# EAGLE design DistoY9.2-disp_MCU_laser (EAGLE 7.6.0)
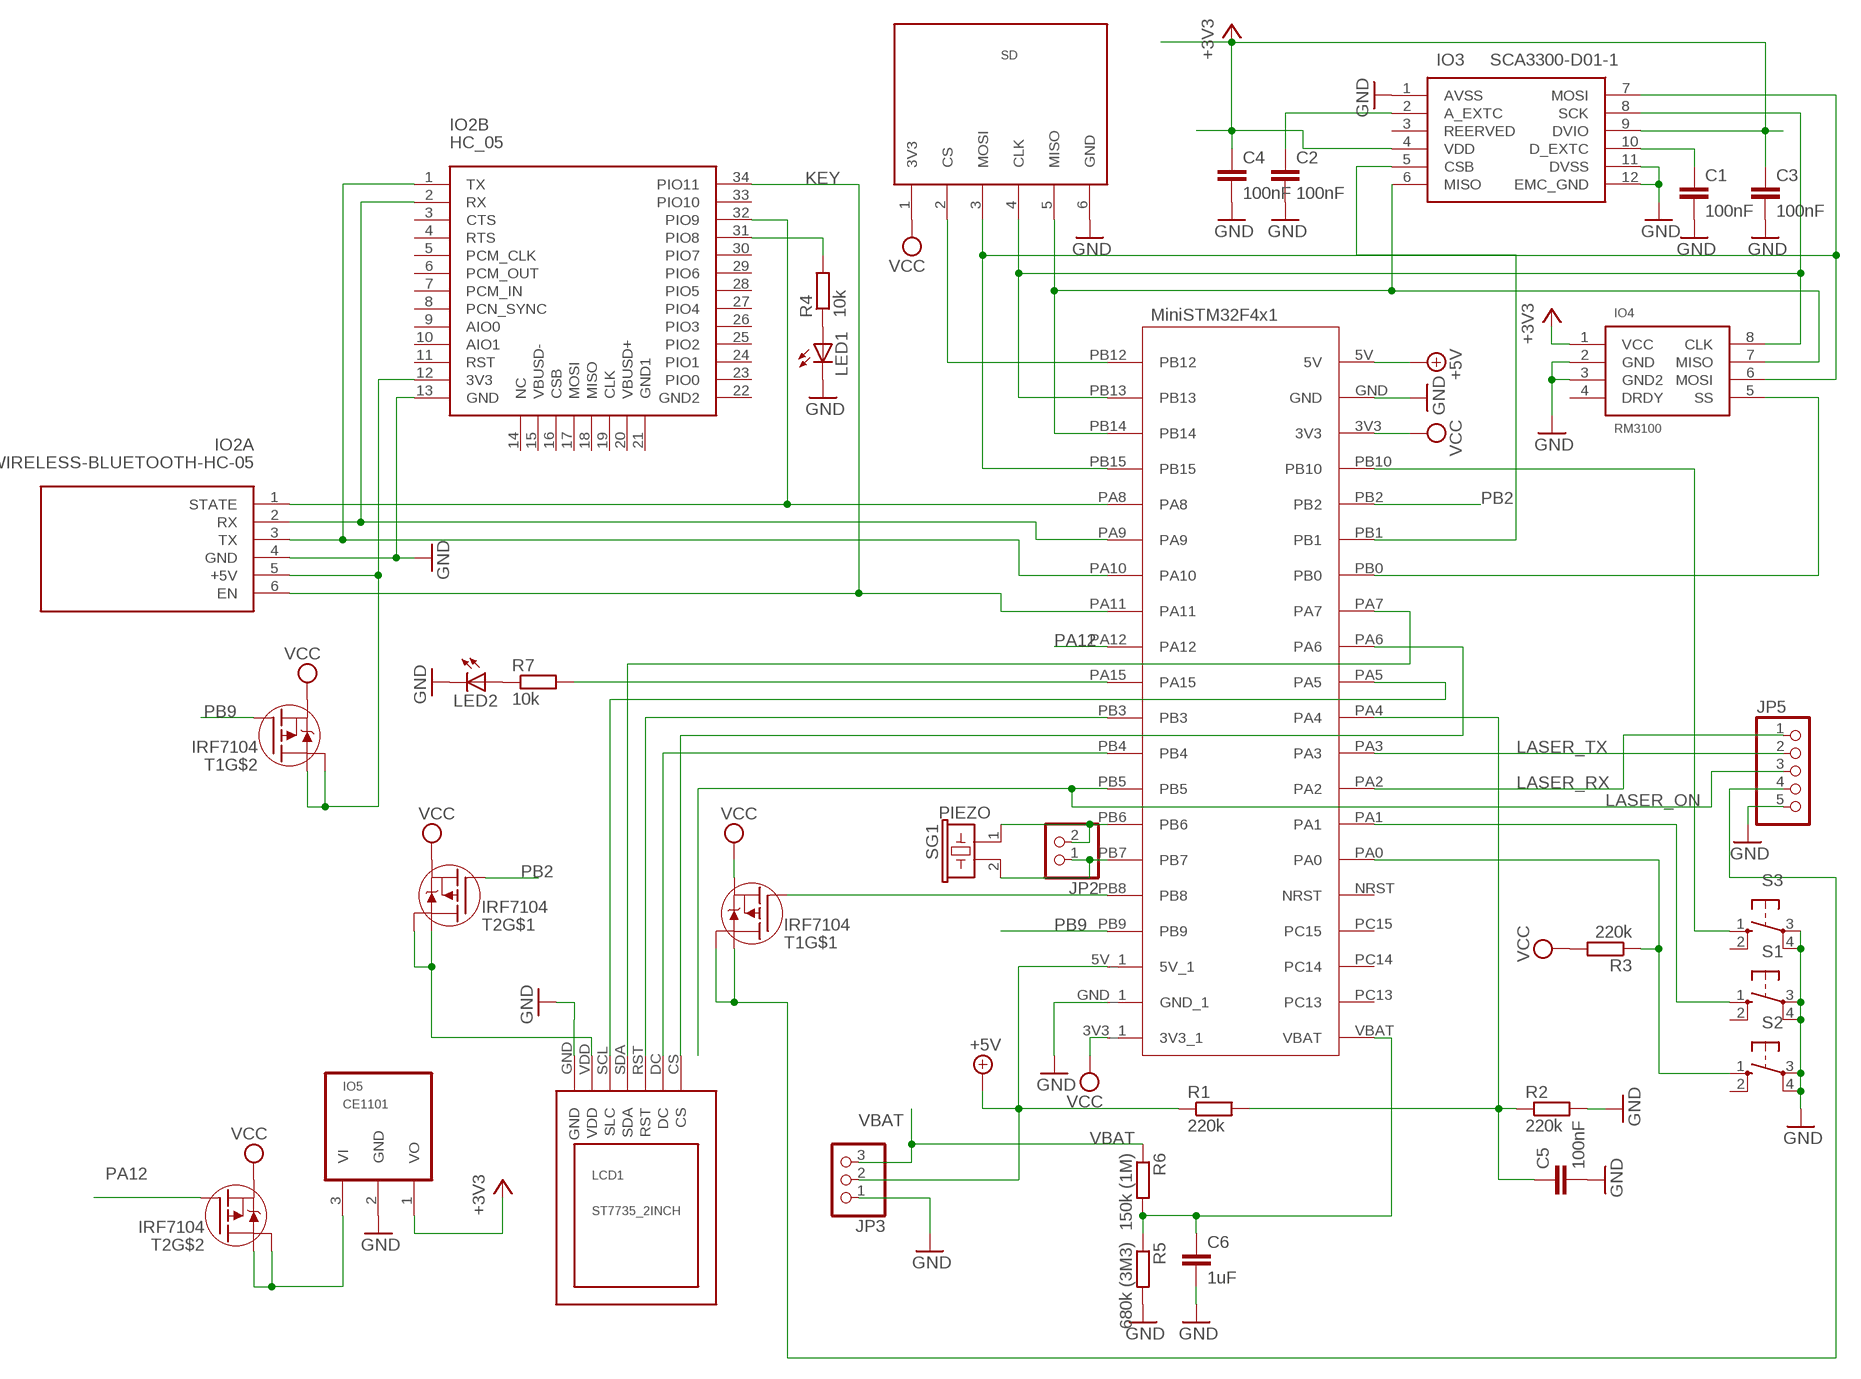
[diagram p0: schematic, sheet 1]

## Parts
C1  100nF  C-EUC0805K  [C0805K]
C2  100nF  C-EUC0805K  [C0805K]
C3  100nF  C-EUC0805K  [C0805K]
C4  100nF  C-EUC0805K  [C0805K]
C5  100nF  C-EUC0805K  [C0805K]
C6  1uF  C-EUC0805K  [C0805K]
IO2A  WIRELESS-BLUETOOTH-HC-05  [WIRELESS-BLUETOOTH-HC-05]
IO2B  HC_05  [BLUETOOTH_SMD]
IO3  SCA3300-D01-1  [SCA3300]
IO4  RM3100  [RM3100]
IO5  CE1101  [CE1101]
JP2  PINHD-1X2/90  [1X02/90]
JP3  PINHD-1X3/90  [1X03/90]
JP5  PINHD-1X5/90  [1X05/90]
LCD1  ST7735_2INCH  [7735_2INCH]
LED1  LEDCHIPLED_0805  [CHIPLED_0805]
LED2  LEDCHIPLED_0805  [CHIPLED_0805]
R1  220k  R-EU_M0805  [M0805]
R2  220k  R-EU_M0805  [M0805]
R3  220k  R-EU_M0805  [M0805]
R4  10k  R-EU_R0805  [R0805]
R5  680k (3M3)  R-EU_M0805  [M0805]
R6  150k (1M)  R-EU_M0805  [M0805]
R7  10k  R-EU_R0805  [R0805]
S1  10-XX  [B3F-10XX]
S2  10-XX  [B3F-10XX]
S3  10-XX  [B3F-10XX]
SD  SD  [SD]
SG1  PIEZO  B/C11L  [B/C11L]
T1  IRF7104  [SO8-2]
T2  IRF7104  [SO8-2]
U$1  STM32F401  [STM32F401]

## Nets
+3V3: C3.1 C4.1 IO3.4(VDD) IO3.9(DVIO) IO4.1(VCC) IO5.1(VO)
+5V: JP3.2 R1.1 U$1.5V U$1.5V_1
GND: C1.2 C2.2 C3.2 C4.2 C5.2 C6.2 IO2A.4(GND) IO2B.13(GND) IO3.1(AVSS) IO3.11(DVSS) IO3.12(EMC_GND) IO4.2(GND) IO4.3(GND2) IO5.2(GND) JP3.1 JP5.5 LCD1.GND LED1.C LED2.C R2.2 R5.2 S1.3(P) S1.4(P1) S2.3(P) S2.4(P1) S3.3(P) S3.4(P1) SD.6(GND) U$1.GND U$1.GND_1
KEY: IO2A.6(EN) IO2B.34(PIO11) U$1.PA11
LASER_ON: JP5.3 U$1.PB5
LASER_RX: JP5.1 U$1.PA2
LASER_TX: JP5.2 U$1.PA3
N$1: IO2A.2(RX) IO2B.2(RX) U$1.PA9
N$2: IO2A.3(TX) IO2B.1(TX) U$1.PA10
N$3: S3.1(S) U$1.PB10
N$4: IO2A.5(+5V) IO2B.12(3V3) T1.5(D) T1.6(D)
N$5: LCD1.SDA U$1.PA7
N$6: LCD1.SCL(SLC) U$1.PA5
N$7: IO2A.1(STATE) IO2B.32(PIO9) U$1.PA8
N$9: C6.1 R5.1 R6.2 U$1.VBAT
N$10: S1.1(S) U$1.PA1
N$11: R3.1 S2.1(S) U$1.PA0
N$12: LCD1.DC U$1.PB4
N$13: LCD1.RST U$1.PB3
N$14: LED2.A R7.1
N$15: T1.2(G) U$1.PB8
N$16: JP5.4 T1.7(D) T1.8(D)
N$17: IO3.6(MISO) IO4.7(MISO) SD.5(MISO) U$1.PB14
N$19: LED1.A R4.1
N$20: IO3.7(MOSI) IO4.6(MOSI) SD.3(MOSI) U$1.PB15
N$21: IO2B.31(PIO8) R4.2
N$22: IO3.8(SCK) IO4.8(CLK) SD.4(CLK) U$1.PB13
N$23: SD.2(CS) U$1.PB12
N$24: C2.1 IO3.2(A_EXTC)
N$25: C1.1 IO3.10(D_EXTC)
N$26: IO4.5(SS) U$1.PB0
N$27: LCD1.VDD T2.7(D) T2.8(D)
N$28: LCD1.CS U$1.PA6
N$29: IO3.5(CSB) U$1.PB1
N$31: JP2.2 SG1.1 U$1.PB6
N$32: JP2.1 SG1.2 U$1.PB7
N$33: C5.1 R1.2 R2.1 U$1.PA4
N$34: R7.2 U$1.PA15
N$35: IO5.3(VI) T2.5(D) T2.6(D)
PA12: T2.4(G) U$1.PA12
PB2: T2.2(G) U$1.PB2
PB9: T1.4(G) U$1.PB9
VBAT: JP3.3 R6.1
VCC: R3.2 SD.1(3V3) T1.1(S) T1.3(S) T2.1(S) T2.3(S) U$1.3V3 U$1.3V3_1
Unconnected: IO2B.3(CTS) IO2B.4(RTS) IO2B.5(PCM_CLK) IO2B.6(PCM_OUT) IO2B.7(PCM_IN) IO2B.8(PCN_SYNC) IO2B.9(AIO0) IO2B.10(AIO1) IO2B.11(RST) IO2B.14(NC) IO2B.15(VBUSD-) IO2B.16(CSB) IO2B.17(MOSI) IO2B.18(MISO) IO2B.19(CLK) IO2B.20(VBUSD+) IO2B.21(GND1) IO2B.22(GND2) IO2B.23(PIO0) IO2B.24(PIO1) IO2B.25(PIO2) IO2B.26(PIO3) IO2B.27(PIO4) IO2B.28(PIO5) IO2B.29(PIO6) IO2B.30(PIO7) IO2B.33(PIO10) IO3.3(REERVED) IO4.4(DRDY) S1.2(S1) S2.2(S1) S3.2(S1) U$1.NRST U$1.PC13 U$1.PC14 U$1.PC15

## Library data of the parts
C1-C6 = rcl:C-EU: CAPACITOR, European symbol
IO2A = diy-modules:WIRELESS-BLUETOOTH-HC-05: Bluetooth Transceiver Module based on HC-05 board Tutorial is available here: https://arduino-info.wikispaces.com/BlueTooth-HC05-HC06-Modules-How-To Click here to find device on ebay.com
IO2B = SerialPortBluetooth:HC_05
IO3 = SCA3300-D01-1:SCA3300-D01-1: Murata SCA3300-D01-1, 3-Axis Accelerometer, +/-1.5 +/-6g, 3 3.6 V, SPI, DFL/SMD 12-Pin Source: Datasheet Check availability; AVAILABILITY: In Stock; DESCRIPTION: Accelerometer X, Y, Z Axis ±1.5g, 3g, 6g - -; MF: Murata Electronics; MP: SCA3300-D01-1; PACKAGE: Nonstandard Murata; PRICE: None; PURCHASE-URL: https://pricing.snapeda.com/search/part/SCA3300-D01-1/?ref=eda
IO4 = SCA3300-D01-1:RM3100
IO5 = SCA3300-D01-1:CE1101
JP2 = pinhead:PINHD-1X2: PIN HEADER
JP3 = pinhead:PINHD-1X3: PIN HEADER
JP5 = pinhead:PINHD-1X5: PIN HEADER
LCD1 = st7735:ST7735_2INCH
LED1 LED2 = led:LED: LED
R1-R7 = rcl:R-EU_: RESISTOR, European symbol
S1-S3 = switch-omron:10-XX: OMRON SWITCH; MPN: B3F-1000; OC_FARNELL: 176432; OC_NEWARK: 36M3542
SD = memory:SD
SG1 = buzzer:B/C11L: BUZZER; OC_FARNELL: unknown; OC_NEWARK: unknown
T1 T2 = irf-2:IRF7104: HEXFET® Power MOSFET Adavanced Process Technology Ultra Low On-Resistance Dual P-Channel MOSFET Surface Mount Available in Tape & Reel Dynamic dv/dt Rating Fast Switching Please connect both Drain-Pins of each FET for thermal Reasons! (Pin 5 with Pin 6, 7 with 8)
U$1 = MiniSTM32F4x1_EAGLE:STM32F401

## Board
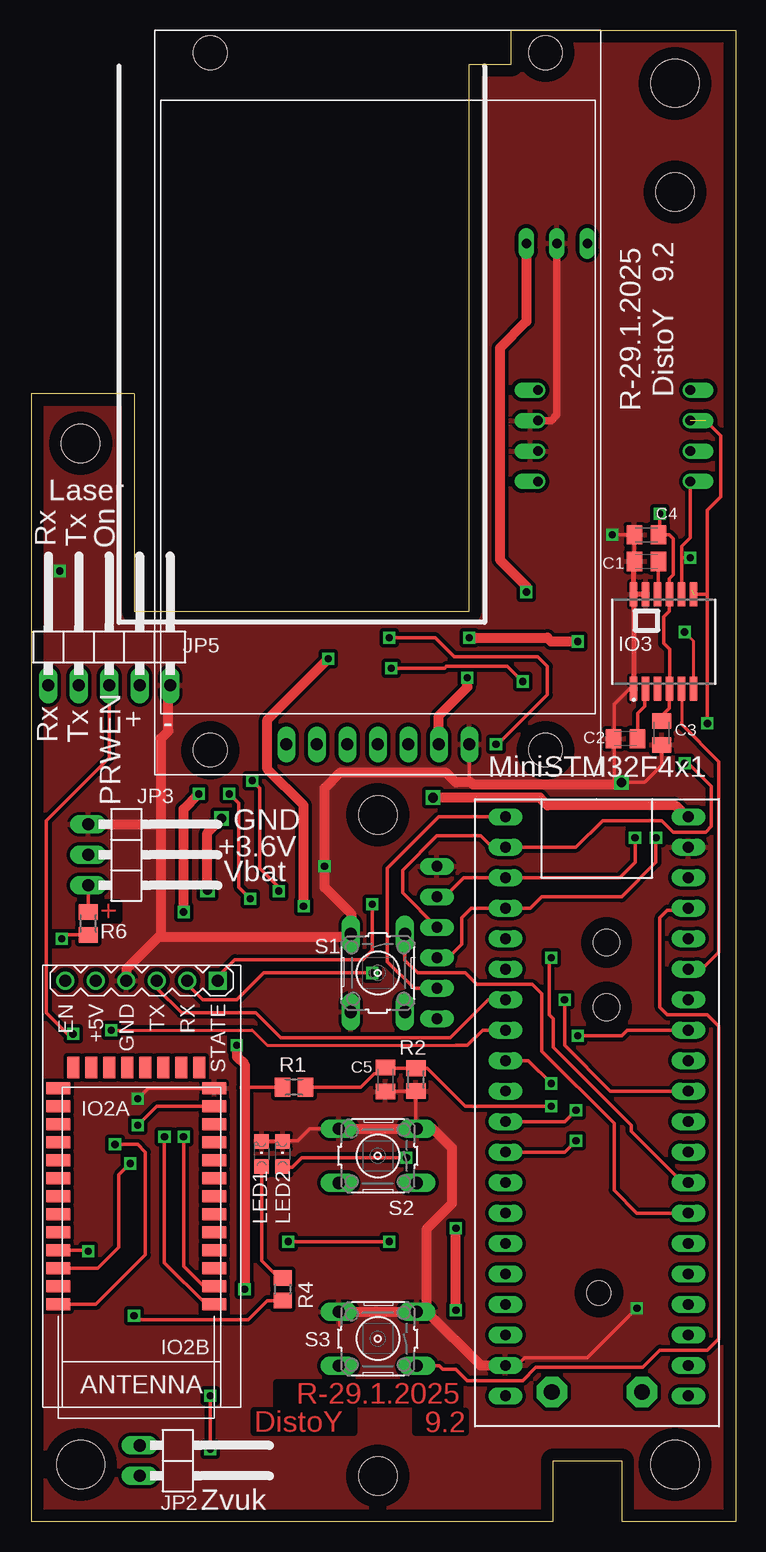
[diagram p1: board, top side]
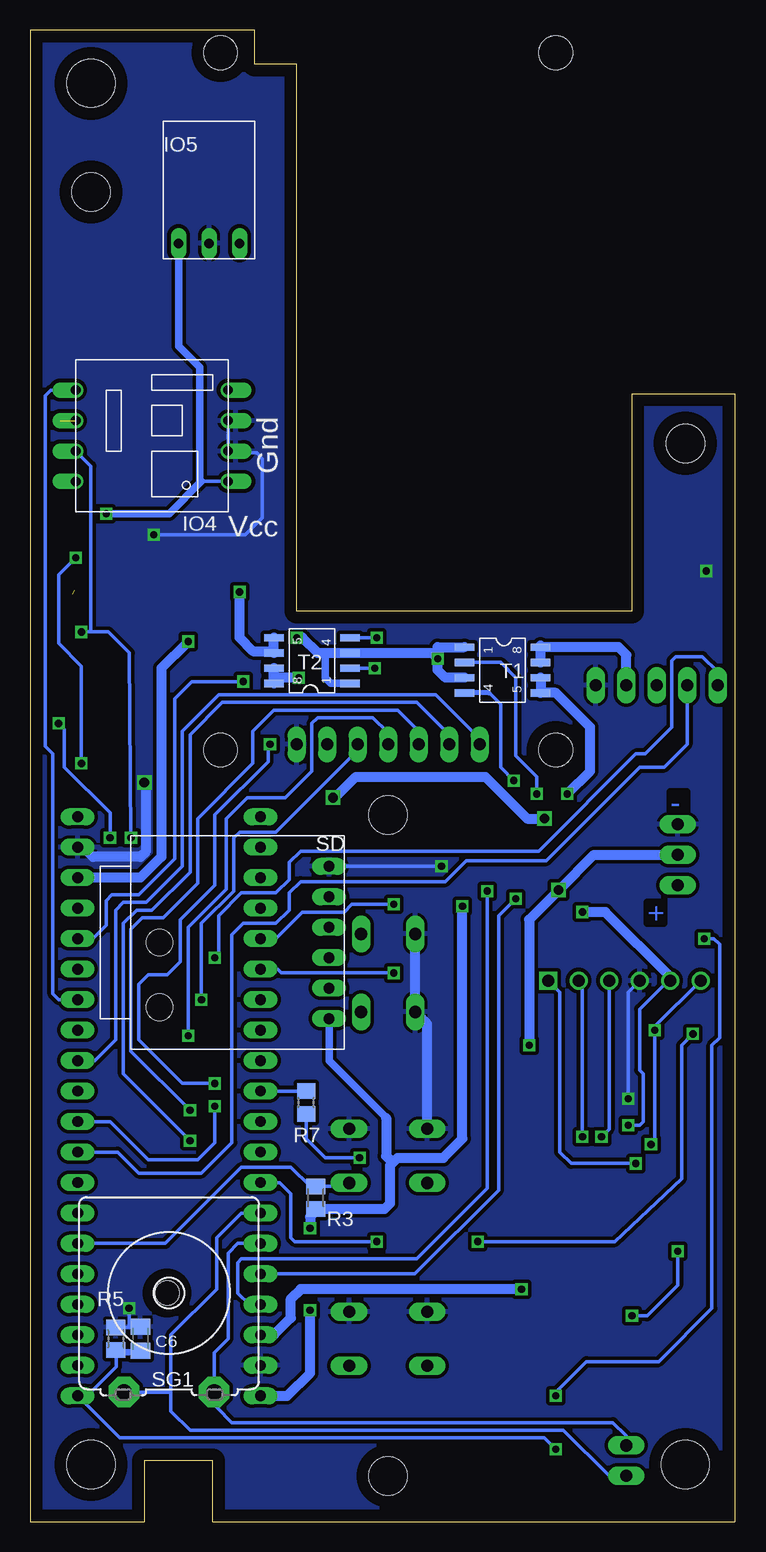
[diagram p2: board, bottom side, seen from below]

Size 58.74 x 124.3 mm. Coordinates in mm from the lower left corner, seen from the top.
Outline: 0,93.98 0,0 43.5,0 43.5,5.08 49.21,5.08 49.21,0 58.74,0 58.74,124.3 40.01,124.3 40.01,121.44 36.51,121.44 36.51,75.88 8.57,75.88 8.57,93.98 0,93.98
Copper layers (1*16): Top 0.035mm / dielectric 1.5mm / Bottom 0.035mm
Design rules "default": minimum track width 10mil, minimum drill 24mil, track to track 8mil, track to pad 8mil, pad to pad 8mil, via to via 8mil, smd to smd 8mil, copper to edge 40mil, drill to drill 8mil, minimum pad ring 10mil, minimum via ring 8mil, stop-mask expansion 4mil, vias tented up to drill 0mil, thermal gap 10mil
Holes 4 mm at 53.66,4.76 4.13,4.76 53.66,119.86
Holes 2 mm at 47.31,19.05
Holes 3.2 mm at 28.89,58.9 28.89,3.81 53.66,110.81 4.13,89.85
Holes 2.2 mm at 47.94,48.26 47.94,42.86

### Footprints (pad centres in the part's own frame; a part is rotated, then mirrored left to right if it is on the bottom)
C0805K = smd 1.3 x 1.6: 1 -1,0; 2 1,0
WIRELESS-BLUETOOTH-HC-05 = drill 1 square: 1 -6.35,-17.145 | drill 1: 2 -3.81,-17.145; 3 -1.27,-17.145; 4 1.27,-17.145; 5 3.81,-17.145; 6 6.35,-17.145
BLUETOOTH_SMD = smd 2 x 1: 1 0,0; 2 0,-1.5; 3 0,-3; 4 0,-4.5; 5 0,-6; 6 0,-7.5; 7 0,-9; 8 0,-10.5; 9 0,-12; 10 0,-13.5; 11 0,-15; 12 0,-16.5; 13 0,-18; 22 13,-18; 23 13,-16.5; 24 13,-15; 25 13,-13.5; 26 13,-12; 27 13,-10.5; 28 13,-9; 29 13,-7.5; 30 13,-6; 31 13,-4.5; 32 13,-3; 33 13,-1.5; 34 13,0 | smd 1 x 1.8: 14 1.25,-19.75; 15 2.75,-19.75; 16 4.25,-19.75; 17 5.75,-19.75; 18 7.25,-19.75; 19 8.75,-19.75; 20 10.25,-19.75; 21 11.75,-19.75
SCA3300 = smd 0.61 x 2: 1 -2.5,-3.935; 2 -1.5,-3.935; 3 -0.5,-3.935; 4 0.5,-3.935; 5 1.5,-3.935; 6 2.5,-3.935; 7 2.5,3.935; 8 1.5,3.935; 9 0.5,3.935; 10 -0.5,3.935; 11 -1.5,3.935; 12 -2.5,3.935
RM3100 = drill 0.8 offset: 1 -6.35,2.54; 2 -6.35,0; 3 -6.35,-2.54; 4 -6.35,-5.08; 5 6.35,-5.08; 6 6.35,-2.54; 7 6.35,0; 8 6.35,2.54
CE1101 = drill 0.8 long: 1 -2.54,-3.81; 2 0,-3.81; 3 2.54,-3.81
1X02/90 = drill 1.016 long: 1 -1.27,-3.81; 2 1.27,-3.81
1X03/90 = drill 1.016 long: 1 -2.54,-3.81; 2 0,-3.81; 3 2.54,-3.81
1X05/90 = drill 1.016 long: 1 -5.08,-3.81; 2 -2.54,-3.81; 3 0,-3.81; 4 2.54,-3.81; 5 5.08,-3.81
7735_2INCH = drill 1 long: CS 7.62,24.765; DC 5.08,24.765; GND -7.62,24.765; RST 2.54,24.765; SCL -2.54,24.765; SDA 0,24.765; VDD -5.08,24.765 | hole 2.8: 13.97,25.241; -13.97,25.241; 13.97,-32.861; -13.97,-32.861
CHIPLED_0805 = smd 1.2 x 1.2: A 0,-1.05; C 0,1.05
M0805 = smd 1.3 x 1.6: 1 -0.95,0; 2 0.95,0
R0805 = smd 1.3 x 1.5: 1 -0.95,0; 2 0.95,0
B3F-10XX = drill 1.016 long: 1 -3.251,2.261; 2 3.251,2.261; 3 -3.251,-2.261; 4 3.251,-2.261
SD = drill 0.9 long: 1 -6.35,-6.35; 2 -3.81,-6.35; 3 -1.27,-6.35; 4 1.27,-6.35; 5 3.81,-6.35; 6 6.35,-6.35
B/C11L = drill 1.321 pad 2.54 octagon: 1 -3.759,-8.255; 2 3.759,-8.255
SO8-2 = smd 0.61 x 1.626: 1 -2.54,-2.54; 2 -1.27,-2.54; 3 0,-2.54; 4 1.27,-2.54; 5 1.27,3.81; 6 0,3.81; 7 -1.27,3.81; 8 -2.54,3.81
STM32F401 = drill 0.9 long: 3V3 7.62,21.59; 3V3_1 -7.62,-21.59; 5V 7.62,26.67; 5V_1 -7.62,-16.51; GND 7.62,24.13; GND_1 -7.62,-19.05; NRST 7.62,-11.43; PA0 7.62,-8.89; PA1 7.62,-6.35; PA2 7.62,-3.81; PA3 7.62,-1.27; PA4 7.62,1.27; PA5 7.62,3.81; PA6 7.62,6.35; PA7 7.62,8.89; PA8 -7.62,16.51; PA9 -7.62,13.97; PA10 -7.62,11.43; PA11 -7.62,8.89; PA12 -7.62,6.35; PA15 -7.62,3.81; PB0 7.62,11.43; PB1 7.62,13.97; PB2 7.62,16.51; PB3 -7.62,1.27; PB4 -7.62,-1.27; PB5 -7.62,-3.81; PB6 -7.62,-6.35; PB7 -7.62,-8.89; PB8 -7.62,-11.43; PB9 -7.62,-13.97; PB10 7.62,19.05; PB12 -7.62,26.67; PB13 -7.62,24.13; PB14 -7.62,21.59; PB15 -7.62,19.05; PC13 7.62,-19.05; PC14 7.62,-16.51; PC15 7.62,-13.97; VBAT 7.62,-21.59

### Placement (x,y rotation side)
C1  51.28,80.01 180 top
C2  49.53,65.25 180 top
C3  52.55,65.72 270 top
C4  51.28,82.23 180 top
C5  29.53,36.83 270 top
C6  49.53,15.24 90 bottom
IO2A  9.21,27.94 180 top
IO2B  15.24,18.1 180 top
IO3  52.7,73.34 0 top
IO4  48.58,89.22 180 bottom
IO5  43.81,110.33 0 bottom
JP2  12.86,5.08 270 top
JP3  8.57,55.56 270 top
JP5  6.51,73.5 0 top
LCD1  28.89,89.53 180 top
LED1  19.21,30.64 0 top
LED2  20.95,30.64 0 top
R1  21.91,36.2 0 top
R2  32.07,36.83 270 top
R3  34.92,26.99 270 bottom
R4  20.95,19.37 270 top
R5  51.59,15.24 90 bottom
R6  4.76,49.85 270 top
R7  35.72,34.92 90 bottom
S1  28.89,45.72 270 top
S2  28.89,30.48 180 top
S3  28.89,15.24 180 top
SD  40.16,48.26 90 bottom
SG1  47.15,19.05 0 bottom
T1  20,70.33 270 bottom
T2  34.61,72.39 90 bottom
U$1  47.15,32.07 0 top

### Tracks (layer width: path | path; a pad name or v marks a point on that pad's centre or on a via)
+3V3  (via drill 0.6)
  Top 0.305: C3.1 52.55,67.15 53.18,67.79 53.18,69.38 IO3.4 53.2,72.68 52.7,73.18 52.7,75.41 53.18,75.88 53.18,77.25 IO3.9 53.18,77.3 53.18,78.58 53.5,78.9 53.5,81.92 53.18,82.23 52.39,82.23 | C4.1 52.39,82.23 | 52.39,82.23 v52.39,83.98
  Bottom 0.305: 44.61,96.36 44.61,96.2 | IO4.1 44.45,86.68
  Bottom 0.61: IO5.1 46.35,97.95 44.61,96.2 44.61,86.84 44.45,86.68 47.15,83.98 v52.39,83.98
+5V  (via drill 0.6, 0.8)
  Top 0.305: R1.1 17.78,36.2
  Top 0.813: v17.15,39.69 17.15,38.73 17.78,38.1 17.78,36.2 v17.78,19.37 | U$1.5V 54.61,58.74 53.66,59.69 43.02,59.69 42.39,60.33 v33.5,60.33 | v14.68,52.63 14.68,57.39 v15.88,58.58
  Bottom 0.813: v17.15,39.69 17.15,50.16 v14.68,52.63 11.75,55.56 JP3.2 | U$1.5V_1 38.42,15.56 36.99,16.99 36.99,18.57 36.2,19.37 v17.78,19.37 | v33.5,60.33 33.34,60.33 31.59,62.07 20.8,62.07 17.3,58.58 v15.88,58.58
GND  (via drill 0.6, 0.8)
  Top 0.305: C5.2 29.58,35.88 R2.2 32.07,32.82 S2.3 | IO2B.13 9.74,36.1 v8.89,35.24 | 25.72,16.35 25.72,17.42 S3.4 | IO3.1 49.88,69.41 48.58,68.1 48.58,65.29 | 48.58,65.29 C2.2 | 48.58,65.29 48.58,61.59 | C1.2 C4.2 v48.42,82.23 | LCD1.GND 36.51,61.75 36.67,61.59 | v50.48,17.78 46.35,13.65 41.12,13.65 40.48,13.02 U$1.GND_1 | S2.4 23.22,32.74 22.22,31.75 21.02,31.75 LED2.C LED1.C | v24.45,54.61 24.77,54.61 24.45,54.29 | C3.2 52.55,63.02 51.12,61.59 v49.21,61.59
  Top 0.406: IO3.11 IO3.12 | IO3.12 IO3.1 | IO3.12 50.2,79.94 C1.2
  Top 0.61: IO5.2 43.81,92.23 43.34,91.76 IO4.3
  Top 0.813: S3.4 28.73,17.5 | 28.73,17.5 S3.3 32.7,17.5 | 28.89,17.34 28.73,17.5 | 32.7,17.5 32.98,17.5 37.46,13.02 U$1.GND_1 | 32.7,17.5 32.98,17.78 32.98,24.41 35.08,26.51 35.08,31.11 33.46,32.74 S2.3 S2.4 | 10.8,58.1 10.8,65.25 11.43,65.88 11.43,69.53 JP5.5 | 10.8,48.74 10.64,48.74 7.94,46.04 IO2A.4 | JP3.1 10.8,58.1 | 10.8,58.1 10.8,48.74 | 10.8,48.74 26.4,48.74 S1.3 26.67,49.01 26.67,50.64 24.45,52.86 24.45,54.29 24.45,61.12 25.72,62.39 34.61,62.39 35.4,61.59 36.67,61.59 36.83,61.44 49.05,61.44 v49.21,61.59
  Bottom 0.305: v8.89,35.24 8.89,44.13 IO2A.4 | C6.2 50.43,16.24 R5.2 50.48,16.19 | 50.48,16.19 49.53,16.19 | IO4.3 IO4.2 42.07,89.06 39.85,89.06 39.37,88.58 39.37,83.66 40.8,82.23 v48.42,82.23 | v50.48,17.78 50.48,16.19 | SD.6 v24.45,54.61
  Bottom 0.813: S2.4 25.64,41.48 S1.4 | 26.67,42.43 S1.4 | v49.21,61.59 49.05,60.96 49.05,55.88 49.53,55.4 53.5,55.4 54.13,56.04 54.61,56.04 U$1.GND | S1.4 S1.3
  other vias: 2.38,79.22
  pour Bottom (isolate 0.305): -0.79,124.62 59.21,124.62 59.37,-0.95 -0.64,-0.95
  pour Top (isolate 0.305): -0.48,124.62 59.21,124.62 59.05,-0.64 -0.64,-0.64
KEY  (via drill 0.6)
  Top 0.254: 6.99,40.96 18.41,40.96 19.68,39.69 35.4,39.69
  Top 0.305: IO2B.34 5.4,18.1 9.52,22.23 9.52,30.8 8.89,31.43 v6.99,31.43 | 35.4,39.69 36.35,39.69 37.62,40.96 U$1.PA11 | 6.99,40.96 v6.67,40.96
  Bottom 0.305: v6.99,31.43 6.67,31.75 6.67,40.48 v6.67,40.96 6.67,41.27 IO2A.6
LASER_ON  (via drill 0.6)
  Top 0.305: JP5.3 6.51,63.66 1.27,58.42 1.27,42.39 3.02,40.64 v3.49,40.64 | v29.84,23.34 v21.43,23.34
  Bottom 0.305: U$1.PB5 37.94,28.26 36.99,27.3 36.99,23.65 36.67,23.34 v29.84,23.34 | v21.43,23.34 10,23.34 4.44,28.57 4.44,39.69 v3.49,40.64
LASER_RX  (via drill 0.6)
  Top 0.305: U$1.PA2 54.29,28.26 50.01,32.54 50.01,33.02 43.5,39.53 43.5,41.91 43.18,42.23 43.18,46.83 v43.34,46.99
  Bottom 0.305: 43.34,47.15 v43.34,46.99 43.02,47.31 43.02,50.48 41.12,52.39 38.26,52.39 37.15,53.5 37.15,54.93 36.2,55.88 16.35,55.88 8.25,63.98 7.46,63.98 5.24,66.2 5.24,71.75 4.92,72.07 2.7,72.07 1.43,70.8 JP5.1
LASER_TX
  Bottom 0.305: U$1.PA3 51.44,30.8 49.69,29.05 44.45,29.05 41.91,31.59 41.91,48.9 40.96,49.85 38.26,49.85 37.15,50.96 37.15,52.39 36.2,53.34 24.13,53.34 22.38,55.09 15.72,55.09 7.94,62.87 5.87,62.87 3.97,64.77 JP5.2
N$1  (via drill 0.6)
  Top 0.305: IO2A.2 13.02,44.77 14.29,43.5 17.15,43.5 19.37,45.72 v28.42,45.72 | IO2B.2 14.38,19.6 12.7,21.27 v12.7,32.07
  Bottom 0.305: v12.7,32.07 12.7,44.77 IO2A.2 | v28.42,45.72 37.78,45.72 38.1,46.04 U$1.PA9
N$2  (via drill 0.6)
  Top 0.305: IO2A.3 10.48,44.45 12.54,42.39 18.73,42.39 20.8,40.32 34.92,40.32 38.1,43.5 U$1.PA10 | IO2B.1 14.6,18.1 11.11,21.59 v11.11,32.07
  Bottom 0.305: IO2A.3 10.48,32.7 v11.11,32.07
N$3
  Top 0.305: S3.1 34.01,12.98 34.29,12.7 35.4,12.7 36.35,11.75 40.96,11.75 42.07,12.86 50.96,12.86 52.39,14.29 56.36,14.29 57.31,15.24 57.31,41.27 56.36,42.23 53.02,42.23 52.39,42.86 52.39,50.32 53.02,50.96 54.61,50.96 U$1.PB10
N$4  (via drill 0.6)
  Top 0.305: IO2B.12 10.47,34.6 v8.89,33.02
  Top 0.813: v12.7,50.8 12.7,59.37 v13.97,60.64
  Bottom 0.305: v8.89,33.02 7.94,33.02 7.62,33.34 7.62,37.31 7.94,37.62 7.94,42.7 5.56,45.09 IO2A.5
  Bottom 0.813: v12.7,50.8 10.8,50.8 5.4,45.4 IO2A.5 | v13.97,60.64 12.07,62.55 12.07,66.2 14.92,69.06 T1.5 T1.6
N$5  (via drill 0.6)
  Top 0.305: U$1.PA7 49.69,40.96 49.21,40.48 v45.56,40.48
  Bottom 0.305: v45.56,40.48 45.56,49.53 42.39,52.7 42.39,58.58 40.64,60.33 37.46,60.33 35.24,62.55 35.24,66.52 34.77,66.99 30.16,66.99 28.89,65.72 LCD1.SDA
N$6  (via drill 0.6)
  Top 0.305: v44.45,43.5 44.45,39.69 48.26,35.88 U$1.PA5
  Bottom 0.305: v44.45,43.5 44.45,49.85 41.75,52.55 41.75,56.99 41.27,57.47 38.26,57.47 31.43,64.29 LCD1.SCL
N$7  (via drill 0.6)
  Top 0.305: IO2B.32 5.54,21.1 7.3,22.86 7.3,28.89 v8.25,29.84 | IO2A.1 15.56,45.4 16.99,46.83 27.62,46.83 28.42,47.62 v28.42,51.44
  Bottom 0.305: v8.25,29.84 13.65,29.84 14.6,30.8 14.6,44.13 IO2A.1 | U$1.PA8 38.26,48.58 36.04,50.8 32.54,50.8 31.91,51.44 v28.42,51.44
N$9  (via drill 0.6)
  Top 0.305: v14.92,6.03 v14.92,10.48 | R6.2 2.86,48.9 v2.54,48.58
  Bottom 0.305: C6.1 50.43,14.24 R5.1 50.48,13.97 51.54,13.97 51.54,12.91 53.98,10.48 U$1.VBAT 51.28,6.99 15.88,6.99 v14.92,6.03 | v14.92,10.48 14.92,10.79 12.38,13.34 6.35,13.34 1.9,17.78 1.9,39.69 1.27,40.32 1.27,48.1 1.75,48.58 v2.54,48.58
N$10
  Top 0.305: S1.1 31.15,46.79 32.23,45.72 36.2,45.72 37.15,44.77 41.75,44.77 42.55,43.97 42.55,39.21 48.58,33.18 48.58,27.62 50.48,25.72 U$1.PA1
N$11
  Bottom 0.305: R3.1 33.66,27.94 33.38,28.22 S2.1 | R3.1 | U$1.PA0 47.47,23.18 41.12,29.53 36.99,29.53 35.4,27.94 R3.1
N$12  (via drill 0.6)
  Top 0.305: v45.4,31.75 44.45,30.8 U$1.PB4
  Bottom 0.305: v45.4,31.75 50.96,37.31 50.96,49.85 49.85,50.96 48.58,50.96 45.4,54.13 45.4,65.56 42.7,68.26 26.51,68.26 23.81,65.56 LCD1.DC
N$13  (via drill 0.6)
  Top 0.305: v45.4,34.29 44.45,33.34 U$1.PB3
  Bottom 0.305: v45.4,34.29 50.32,39.21 50.32,49.37 49.37,50.32 47.63,50.32 44.77,53.18 44.77,58.58 40.16,63.18 40.16,65.88 38.42,67.63 28.1,67.63 26.35,65.88 LCD1.RST
N$14  (via drill 0.6)
  Top 0.305: v31.27,30.32 22.54,30.32 21.75,29.53 21.02,29.53 LED2.A
  Bottom 0.305: R7.1 35.72,31.91 34.13,30.32 v31.27,30.32
N$15  (via drill 0.6)
  Top 0.305: v16.51,60.64 17.3,59.85 17.3,52.86 v18.26,51.91
  Bottom 0.305: T1.2 19.53,71.6 18.26,70.33 18.26,63.82 16.51,62.07 v16.51,60.64 | U$1.PB8 26.67,20.64 19.68,27.62 19.68,50.48 v18.26,51.91
N$16
  Bottom 0.813: JP5.4 9.05,72.23 9.68,72.87 T1.8 T1.7 16.19,73.03
N$17  (via drill 0.6)
  Top 0.254: IO3.6 55.2,73.38 v54.45,74.14
  Top 0.305: SD.5 34.45,52.07 36.04,53.66 U$1.PB14 49.05,53.66 50.32,54.93 v50.32,56.99
  Bottom 0.305: v50.32,56.99 50.46,72.39 52.21,74.14 53.5,74.14 | IO4.7 53.66,87.95 53.66,74.3 53.5,74.14 | v54.45,74.14 53.5,74.14
N$19
  Top 0.305: R4.1 20.64,20.32 19.21,21.75 LED1.A
N$20  (via drill 0.6)  (2 unrouted)
  Top 0.305: 55.05,77.59 55.09,77.63 | SD.3 34.77,46.99 35.88,48.1 35.88,50.32 36.67,51.12 U$1.PB15 41.59,51.12 42.55,52.07 49.21,52.07 52.07,54.93 v52.07,56.99 | v56.36,66.52 56.36,77.15 | 56.36,77.15 56.36,84.3 57.47,85.41 57.47,90.49 56.2,91.76 | 56.36,77.15 56.23,77.28 IO3.7
  Bottom 0.305: v52.07,56.99 52.07,59.05 55.88,62.87 55.88,66.04 v56.36,66.52
N$21  (via drill 0.6)
  Top 0.305: IO2B.31 4.71,22.6 v4.76,22.54 | v8.57,17.14 8.89,16.83 18.1,16.83 19.68,18.41 R4.2
  Bottom 0.305: v4.76,22.54 4.76,19.68 7.3,17.14 v8.57,17.14
N$22  (via drill 0.6)
  Top 0.305: SD.4 30.96,52.39 30.96,54.29 33.81,57.15 37.46,57.15 38.42,56.2 U$1.PB13 45.4,56.2 47.63,58.42 52.55,58.42 53.5,57.47 56.2,57.47 56.67,57.94 56.67,61.28 54.77,63.18 v54.45,63.18 | IO3.8 54.2,80.33 | 54.2,80.33 54.2,81.28 54.93,82 IO4.8 54.61,87 | v54.93,80.33 54.2,80.33
  Bottom 0.305: v54.45,63.18 54.45,71.28 56.36,73.18 56.36,78.9 v54.93,80.33
N$23
  Top 0.305: SD.2 31.91,44.45 29.69,46.67 29.69,54.45 33.97,58.74 U$1.PB12
N$24
  Top 0.305: C2.1 50.53,67.36 51.12,67.94 51.12,69.32 IO3.2
N$25
  Top 0.305: C1.1 52.28,77.35 IO3.10
N$26
  Bottom 0.305: IO4.5 56.99,94.3 57.47,93.82 57.47,64.61 56.83,63.98 56.83,43.97 56.36,43.5 U$1.PB0
N$27  (via drill 0.6)
  Top 0.813: LCD1.VDD 33.97,67.15 36.35,69.53 v36.35,70.33
  Bottom 0.813: T2.8 38.42,70.33 | T2.7 38.42,70.48 38.42,70.33 | v36.35,70.33 38.42,70.33
N$28
  Bottom 0.305: U$1.PA6 53.34,38.42 51.59,40.16 51.59,50.96 50.96,51.59 49.05,51.59 46.04,54.61 46.04,65.88 43.02,68.9 24.92,68.9 21.27,65.25 LCD1.CS
N$29
  Top 0.254: IO3.5 54.2,66.6
  Top 0.305: 54.2,66.6 54.2,66.44 57.31,63.34 57.31,47.47 55.88,46.04 U$1.PB1
N$31
  Bottom 0.305: JP2.2 10.48,3.81 14.29,7.62 45.4,7.62 46.99,9.21 46.99,10.79 | 46.99,10.79 46.99,15.56 43.18,19.37 43.18,23.65 41.12,25.72 U$1.PB6 | SG1.1 46.99,10.79
N$32
  Bottom 0.305: JP2.1 9.05,7.14 10.16,8.26 41.91,8.26 43.18,9.53 43.18,10.59 SG1.2 43.39,14.08 42.23,15.24 42.23,22.38 41.43,23.18 U$1.PB7
N$33  (via drill 0.6)
  Top 0.305: 29.16,37.47 C5.1 | 29.16,37.47 29.21,37.47 29.53,37.78 R2.1 33.02,37.78 36.2,34.61 v43.34,34.61 | R1.2 27.46,36.2 28.57,37.31 29,37.31 29.16,37.47
  Bottom 0.305: U$1.PA4 52.07,33.34 48.89,30.16 44.77,30.16 43.34,31.59 v43.34,34.61
N$34
  Bottom 0.305: R7.2 U$1.PA15
N$35  (via drill 0.6)
  Top 0.813: IO5.3 41.27,100.01 39.05,97.79 39.05,80.17 41.27,77.95 v41.27,77.47
  Bottom 0.305: 38.74,72.55 38.58,72.55 T2.6
  Bottom 0.813: T2.6 T2.5 | 38.74,72.55 40.16,72.55 41.27,73.66 v41.27,77.47
PA12  (via drill 0.6)
  Top 0.305: U$1.PA12 41.43,38.42 v43.34,36.51 | v38.74,64.77 38.89,64.77 43.02,68.9 43.02,71.28 42.23,72.07 35.24,72.07 33.66,73.66 v29.84,73.66
  Bottom 0.305: v43.34,36.51 46.04,36.51 49.69,40.16 49.69,44.77 48.89,45.56 47.31,45.56 46.2,46.67 46.2,50.16 43.34,53.02 43.34,58.9 38.89,63.34 38.89,64.61 v38.74,64.77 | v29.84,73.66 T2.4
PB2  (via drill 0.6)
  Top 0.305: v30,71.12 34.45,71.12 34.61,71.28 39.69,71.28 v40.96,70.01
  Bottom 0.305: U$1.PB2 53.5,48.58 52.39,49.69 52.39,51.75 51.91,52.23 49.69,52.23 46.67,55.24 46.67,68.58 45.24,70.01 v40.96,70.01 | T2.2 v30,71.12
PB9  (via drill 0.6)
  Top 0.305: v18.41,61.75 19.05,61.12 19.05,54.45 20.64,52.86 v20.64,52.55
  Bottom 0.305: 20.48,69.06 19.53,68.1 19.53,62.87 v18.41,61.75 | U$1.PB9 40.48,18.1 41.43,19.05 41.43,21.59 41.12,21.91 26.51,21.91 20.64,27.78 v20.64,52.55
  Bottom 0.406: 20.48,69.06 T1.4
VBAT
  Top 0.305: R6.1 JP3.3
VCC  (via drill 0.6)
  Top 0.813: v35.4,17.62 v35.4,24.45 | v22.7,51.28 22.7,59.69 19.68,62.71 19.68,66.83 v24.77,71.91 | v45.56,73.34 43.34,73.34 43.02,73.66 v36.51,73.66
  Bottom 0.305: R3.2 34.85,25.96
  Bottom 0.61: SD.1 33.81,38.42 29.05,33.66 | T2.1 33.66,69.85 34.13,70.33 34.13,72.39
  Bottom 0.813: v35.4,17.62 35.4,12.38 37.31,10.48 U$1.3V3_1 | v35.4,24.45 35.4,25.4 34.85,25.96 34.77,26.04 29.21,26.04 28.73,26.51 28.73,29.69 28.5,29.92 | 28.5,29.92 28.1,30.32 24.29,30.32 22.7,31.91 v22.7,51.28 | 29.05,33.66 29.05,30.48 28.5,29.92 | T1.1 24.77,72.87 v24.77,71.91 | T1.3 24.13,70.33 24.77,70.96 v24.77,71.91 | U$1.3V3 49.53,53.66 47.78,55.4 47.78,71.12 v45.56,73.34 | v24.77,71.91 25.24,72.39 T2.3 34.13,72.39 34.77,72.39 36.04,73.66 v36.51,73.66

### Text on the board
Top: + | R-29.1.2025 | 9.2 | DistoY
Bottom: - | +
tPlace: 9.2 | DistoY | R-29.1.2025 | Laser | Rx | Tx | On | + | - | Rx | Tx | PRWEN | GND | +3.6V | Vbat | Zvuk
bPlace: Gnd | Vcc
